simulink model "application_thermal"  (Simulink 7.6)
settings: Solver=ode15s  StartTime=0.0  StopTime=2.5  RelTol=1e-3
InitFcn:
  | Tinf=100+273.15;
  | r=0.05; % rayon
  | l=1e-2 % longueur du cylindre
  | A=2*pi*r^2+2*pi*r*l; % surface d'échange
  | h=400; % coefficient d'échange
  | Cp=444; % capacité calorifique
  | m=5e-3; % masse du cylindre
  | V=(pi*r^2*l);
  | rho=m/V; % masse volumique
  | T0=20+273.15; % température initiale
  | 
  | % Constante de temps
  | R=1/(h*A);
  | C=rho*Cp*V;
  | tau=R*C;
StopFcn:
  | close all
  | load temperatures.mat
  | plot(x(1,:), x(3,:))
  | title('\theta(t)/\theta0')
  | grid
  | xlabel('temps')
  | figure
  | plot(x(1,:), x(4,:),x(1,:), x(5,:))
  | 
  | grid
  | %axis([0 6000 -5 120])
  | title('Tranferts convectif, conductif et masse thermique')
  | xlabel('temps')
libraries: fl_lib x8, nesl_utility x4

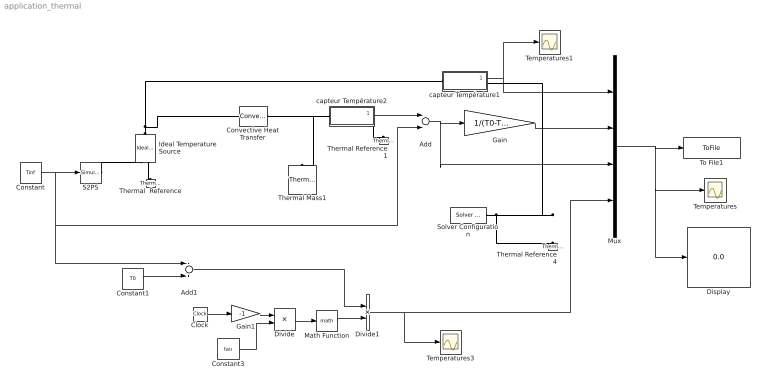
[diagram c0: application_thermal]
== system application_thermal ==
  Add : Sum  Inputs=+-
  Add1 : Sum  Inputs=-+
  Clock : Clock
  Constant : Constant  Value=Tinf
  Constant1 : Constant  Value=T0
  Constant3 : Constant  Value=tau
  Convective Heat Transfer : fl_lib/Thermal/Thermal Elements/Convective Heat Transfer  DialogController=NetworkEngine.DynNeDlgSource  SystemSampleTime=-1  area=A m^2  heat_tr_coeff=h W/(m^2 * K)  Q_Log=off  T_Log=off  LocalVarNames=|heat_flow|temperature_diff  LocalVarDescs=|Heat flow (J/s)|Temperature difference (K)  LocalVarLogging=[0 0]
  Display : Display
  Divide : Product  Inputs=*/
  Divide1 : Product  Inputs=**
  Gain : Gain  Gain=1/(T0-Tinf)
  Gain1 : Gain  Gain=-1
  Ideal Temperature Source : fl_lib/Thermal/Thermal Sources/Ideal Temperature Source  DialogController=NetworkEngine.DynNeDlgSource  SystemSampleTime=-1  Q_Log=off  T_Log=off  LocalVarNames=|Q|T  LocalVarDescs=|Q|T  LocalVarLogging=[0 0]
  Math Function : Math
  Mux : Mux
  S2PS : nesl_utility/Simulink-PS Converter  DialogController=NetworkEngine.DynNeUtilDlgSource  SystemSampleTime=-1  PhysicalDomain=network_engine_domain  LeftPortType=input  RightPortType=output  SubClassName=ps_input  Unit=1  AffineConversion=off  InputFilterTimeConstant=.001  UdotUserProvided=0
  Solver Configuration : nesl_utility/Solver Configuration  DialogController=NetworkEngine.DynNeUtilDlgSource  SystemSampleTime=-1  PhysicalDomain=network_engine_domain  LeftPortType=input  RightPortType=generic  SubClassName=solver  Accelerate=off  Profile=off  ResidualTolerance=1e-9  MaxNonlinIter=12  MaxModeIter=2  DoFixedCost=off  UseLocalSampling=off  DoDC=off  LinearAlgebra=Sparse  LocalSolverSampleTime=.001  LocalSolverChoice=NE_BACKWARD_EULER_ADVANCER  UseLocalSolver=off
  Temperatures : Scope
  Temperatures1 : Scope
  Temperatures3 : Scope
  Thermal  Reference : fl_lib/Thermal/Thermal Elements/Thermal Reference  DialogController=NetworkEngine.DynNeDlgSource  SystemSampleTime=-1  Q_Log=off  LocalVarNames=|Q  LocalVarDescs=|Q  LocalVarLogging=[]
  Thermal Mass1 : fl_lib/Thermal/Thermal Elements/Thermal Mass  DialogController=NetworkEngine.DynNeDlgSource  SystemSampleTime=-1  mass=m kg  sp_heat=Cp J/kg/K  init_temp=T0 K  Q_Log=off  LocalVarNames=|heat_flow|temperature  LocalVarDescs=|Heat flow (J/s)|Mass temperature (K)  LocalVarLogging=[0 0]
  Thermal Reference1 : fl_lib/Thermal/Thermal Elements/Thermal Reference  DialogController=NetworkEngine.DynNeDlgSource  SystemSampleTime=-1  Q_Log=off  LocalVarNames=|Q  LocalVarDescs=|Q  LocalVarLogging=[]
  Thermal Reference4 : fl_lib/Thermal/Thermal Elements/Thermal Reference  DialogController=NetworkEngine.DynNeDlgSource  SystemSampleTime=-1  Q_Log=off  LocalVarNames=|Q  LocalVarDescs=|Q  LocalVarLogging=[]
  To File1 : ToFile  Filename=temperatures  MatrixName=x
  capteur Température1 : Subsystem
  capteur Température2 : Subsystem
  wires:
  Constant/1 -> S2PS/1, Add/2, Add1/1
  capteur Température1/1(T) -> Mux/1, Temperatures1/1
  Mux/1 -> To File1/1, Temperatures/1, Display/1
  Add/1 -> Gain/1, Mux/3
  Gain/1 -> Mux/2
  capteur Température2/1(T) -> Add/1
  Clock/1 -> Gain1/1
  Gain1/1 -> Divide/1
  Constant3/1 -> Divide/2
  Divide/1 -> Math Function/1
  Math Function/1 -> Divide1/2
  Divide1/1 -> Temperatures3/1, Mux/4
  Constant1/1 -> Add1/2
  Add1/1 -> Divide1/1
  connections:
  capteur Température2/LConn1 -- Convective Heat Transfer/RConn1 -- Thermal Mass1/LConn1
  Ideal Temperature Source/RConn2 -- Thermal  Reference/LConn1
  Ideal Temperature Source/LConn1 -- capteur Température1/LConn1 -- Convective Heat Transfer/LConn1
  Solver Configuration/RConn1 -- Thermal Reference4/LConn1 -- capteur Température1/RConn1
  S2PS/RConn1 -- Ideal Temperature Source/RConn1
  capteur Température2/RConn1 -- Thermal Reference1/LConn1

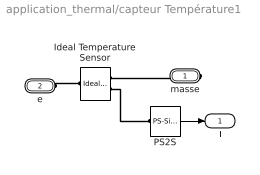
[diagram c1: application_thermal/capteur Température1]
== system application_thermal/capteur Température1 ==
  Ideal Temperature Sensor : fl_lib/Thermal/Thermal Sensors/Ideal Temperature Sensor  DialogController=NetworkEngine.DynNeDlgSource  SystemSampleTime=-1  Qs_Log=off  Ts_Log=off  LocalVarNames=|Qs|Ts  LocalVarDescs=|Qs|Ts  LocalVarLogging=[0 0]
  PS2S : nesl_utility/PS-Simulink Converter  DialogController=NetworkEngine.DynNeUtilDlgSource  SystemSampleTime=-1  PhysicalDomain=network_engine_domain  LeftPortType=input  RightPortType=output  SubClassName=ps_output  Unit=1  AffineConversion=off
  masse : PMIOPort  Port=1  Side=Right
  e : PMIOPort  Port=2  Side=Left
  T : Outport
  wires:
  PS2S/1 -> T/1
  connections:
  Ideal Temperature Sensor/RConn2 -- PS2S/LConn1
  masse/RConn1 -- Ideal Temperature Sensor/RConn1
  e/RConn1 -- Ideal Temperature Sensor/LConn1

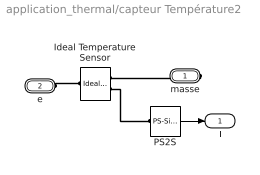
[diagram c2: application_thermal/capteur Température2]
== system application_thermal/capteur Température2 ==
  Ideal Temperature Sensor : fl_lib/Thermal/Thermal Sensors/Ideal Temperature Sensor  DialogController=NetworkEngine.DynNeDlgSource  SystemSampleTime=-1  Qs_Log=off  Ts_Log=off  LocalVarNames=|Qs|Ts  LocalVarDescs=|Qs|Ts  LocalVarLogging=[0 0]
  PS2S : nesl_utility/PS-Simulink Converter  DialogController=NetworkEngine.DynNeUtilDlgSource  SystemSampleTime=-1  PhysicalDomain=network_engine_domain  LeftPortType=input  RightPortType=output  SubClassName=ps_output  Unit=1  AffineConversion=off
  masse : PMIOPort  Port=1  Side=Right
  e : PMIOPort  Port=2  Side=Left
  T : Outport
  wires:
  PS2S/1 -> T/1
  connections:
  e/RConn1 -- Ideal Temperature Sensor/LConn1
  masse/RConn1 -- Ideal Temperature Sensor/RConn1
  Ideal Temperature Sensor/RConn2 -- PS2S/LConn1
